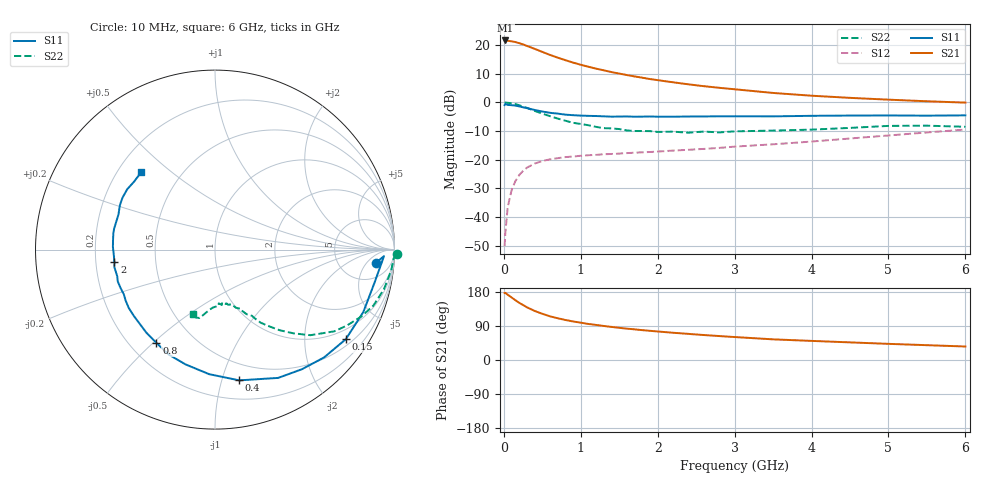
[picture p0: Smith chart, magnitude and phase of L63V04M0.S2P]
!  INFINEON TECHNOLOGIES Small Signal Semiconductors
! BFR380L3 , Si-NPN RF-Transistor in TSLP-3-1
!  Vce=3 V,  Ic=4 mA
! Common Emitter S-Parameters:  07. March 2005
#  GHz  S  MA  R  50
! f  S11  S21  S12  S22
! GHz  Mag  Ang  Mag  Ang  Mag  Ang  Mag  Ang
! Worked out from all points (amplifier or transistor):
!   36 points, 10 MHz to 6 GHz, reference 50 ohm
!   highest |S21| = 21.7 dB at 20 MHz (marker M1)
!   |S21| within 3 dB of that: start of sweep to 407.4 MHz
!   unconditionally stable (mu >= 1): 2.499 GHz to 4.675 GHz
!   at 250 MHz: K = 0.14, MSG = 22.1 dB, |S12| = -23.9 dB
!   at 1.4 GHz: K = 0.71, MSG = 14.3 dB, |S12| = -18.0 dB
!   at 6 GHz: K = 0.92, MSG = 4.7 dB, |S12| = -9.4 dB
!   S11 on the Smith chart (normalised r, x): 10 MHz: 12, -9; 150 MHz: 0.68, -3.09; 400 MHz: 0.35, -1.14; 800 MHz: 0.31, -0.51; 2 GHz: 0.28, -0.06; 6 GHz: 0.30, +0.40
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0.01  0.8999 -4.7  12.05 176.8  0.0031 84.2  1.013 -1.4
0.02  0.9423 -2.2  12.1 177.2  0.0054 91.2  0.9969 -2.8
0.05  0.9075 -11.8  11.95 172.4  0.0148 86.1  0.9886 -6.7
0.1  0.8966 -22.8  11.69 165.1  0.0292 78.7  0.967 -13.2
0.15  0.8834 -34.4  11.35 157.8  0.0424 72.2  0.9359 -19.5
0.2  0.8545 -44.7  10.86 150.9  0.054 67.2  0.8961 -24.6
0.25  0.8238 -54.0  10.31 145.1  0.064 62.4  0.8483 -29.9
0.3  0.7967 -63.8  9.728 139.1  0.0728 58.9  0.806 -34.4
0.4  0.741 -79.5  8.646 129.5  0.0857 51.9  0.7141 -41.9
0.5  0.6948 -92.7  7.641 121.9  0.0952 47.5  0.6386 -46.9
0.6  0.6601 -104.5  6.767 115.3  0.1017 44.1  0.5769 -51.2
0.8  0.6138 -122.1  5.479 105.6  0.1113 40.1  0.4803 -58.0
0.9  0.6001 -129.7  4.969 101.7  0.1139 39.1  0.4418 -60.0
1.1  0.584 -140.7  4.201 95.1  0.12 38.5  0.4008 -63.9
1.5  0.5681 -158.1  3.198 84.9  0.1282 39.8  0.3437 -70.3
2  0.5648 -172.9  2.453 75.3  0.1389 43.1  0.3061 -78.0
2.2  0.5645 -177.0  2.25 71.9  0.1447 44.8  0.3094 -78.4
2.8  0.5737 170.9  1.804 63.2  0.1611 50.3  0.3001 -86.0
3.5  0.5723 160.0  1.467 54.5  0.1862 54.6  0.3231 -92.1
4.5  0.591 150.7  1.204 46.5  0.2351 60.5  0.3599 -98.8
5.5  0.5888 139.9  1.05 39.1  0.2996 62.0  0.3937 -105.4
6  0.5959 133.6  0.995 35.6  0.3371 61.4  0.3766 -108.8
